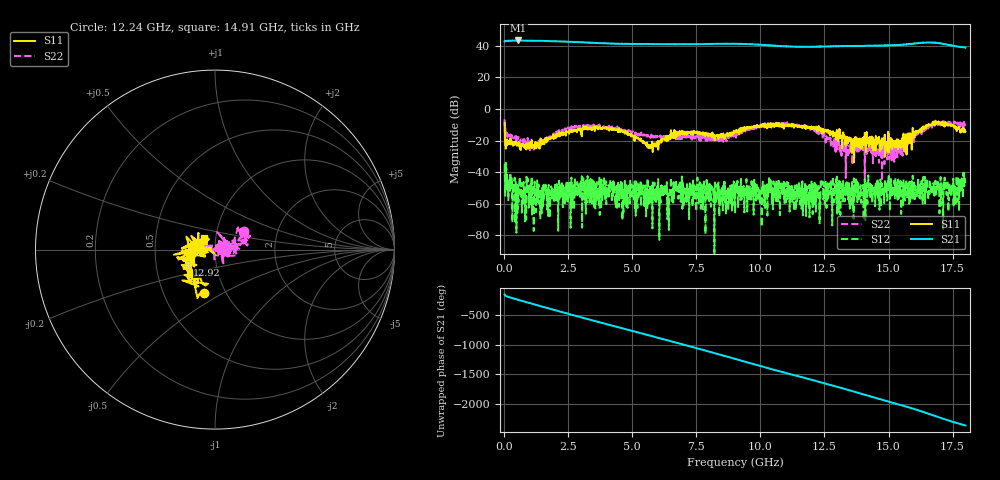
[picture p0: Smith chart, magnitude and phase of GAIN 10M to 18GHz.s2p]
!Agilent Technologies,E8361C,US49010292,A.09.42.06
!Agilent E8361C: A.09.42.06
!Date: Wednesday, May 21, 2025 00:39:04
!Correction: S11(Full 2 Port(1,2))
!S21(Full 2 Port(1,2))
!S12(Full 2 Port(1,2))
!S22(Full 2 Port(1,2))
!S2P File: Measurements: S11, S21, S12, S22:
# Hz S  dB  R 50
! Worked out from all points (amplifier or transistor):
!   1600 points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, 21.24 MHz to 18 GHz, reference 50 ohm
!   highest |S21| = 43.3 dB at 549.7 MHz (marker M1)
!   |S21| within 3 dB of that: start of sweep to 10.22 GHz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
!   unconditionally stable (mu >= 1): 1.078 GHz to 2.629 GHz; 4.261 GHz to 10.71 GHz; 10.72 GHz to 15.94 GHz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
!   at 3.012 GHz: K = 1.26, MAG = 42.6 dB, |S12| = -49.3 dB
!   at 9.016 GHz: K = 7.73, MAG = 41.4 dB, |S12| = -65.4 dB
!   at 18 GHz: K = 1.26, MAG = 39.7 dB, |S12| = -46.8 dB
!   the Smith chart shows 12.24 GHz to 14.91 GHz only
!   S11 on the Smith chart (normalised r, x): 12.24 GHz: 0.79, -0.41; 12.92 GHz: 0.73, -0.12; 14.91 GHz: 0.88, +0.12
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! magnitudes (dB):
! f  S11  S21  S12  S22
! 21.24 MHz  -8.7  42.6  -35.1  -6.5
! 234.9 MHz  -21.7  43.1  -51.0  -16.9
! 549.7 MHz  -21.4  43.3  -47.9  -18.0
! 1.202 GHz  -24.6  43.0  -54.8  -24.5
! 3.023 GHz  -12.6  42.1  -52.0  -10.7
! 6.014 GHz  -25.8  40.9  -44.3  -17.8
! 6.205 GHz  -19.0  40.9  -48.8  -17.4
! 6.464 GHz  -18.3  40.9  -50.6  -17.4
! 6.7 GHz  -14.3  40.9  -47.0  -18.1
! 7.768 GHz  -14.7  41.0  -48.0  -17.2
! 9.016 GHz  -14.4  41.2  -65.4  -16.6
! 10.42 GHz  -9.8  40.1  -52.6  -10.0
! 12.01 GHz  -12.0  39.3  -58.9  -12.4
! 12.24 GHz  -12.0  39.4  -54.7  -14.2
! 12.92 GHz  -15.2  39.6  -51.3  -26.4
! 13.38 GHz  -20.2  39.8  -54.3  -29.1
! 14.91 GHz  -21.0  40.2  -50.2  -25.4
! 15.01 GHz  -16.1  40.2  -42.4  -24.3
! 15.64 GHz  -21.9  40.7  -57.9  -23.3
! 16.82 GHz  -8.8  41.9  -52.2  -8.9
! 17.66 GHz  -14.0  39.5  -43.9  -8.8
! 18 GHz  -14.3  38.7  -46.8  -10.5
